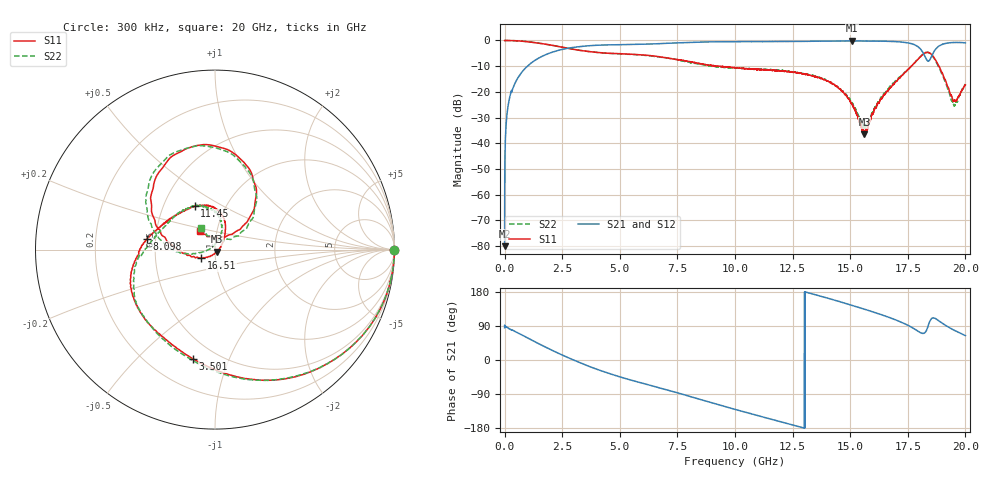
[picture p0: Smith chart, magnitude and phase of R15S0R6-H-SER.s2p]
!{R15S0R6}
!Johanson Technology Inc.
!www.johansontechnology.com
!Test Board Conditions:
!Substrate Type  RO4350B
!Substrate Thickness  20 mil
!Substrate Dk  3.66
!TL Type: GCPW
!TL Trace Width  34 mil
!TL Gap  10 mil
!Electrode orientation  Horizontal
!DUT TOPOLOGY	SERIES
!Mounting Pad LxW  26x52 mil
! Created Sat Feb  6 12:07:06 2021
# hz S ma R 50
! 2 Port Network Data from SP1.SP block
! freq  magS11  angS11  magS21  angS21  magS12  angS12  magS22  angS22
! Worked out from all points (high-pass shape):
!   20001 points, 300 kHz to 20 GHz, reference 50 ohm
!   highest |S21| = -0.15 dB at 15.06 GHz (marker M1); lowest = -80.1 dB at 300 kHz (marker M2)
!   |S21| within 3 dB of the highest: 2.681 GHz to 18.03 GHz (15.35 GHz wide, 148 % of centre); 18.73 GHz to end of sweep
!   lowest |S11| = -36.5 dB at 15.62 GHz (marker M3), VSWR 1.03, Z = 51 - j1.11 ohm
!   |S11| at or under -10 dB: 9.237 GHz to 9.311 GHz (73.82 MHz wide, 0.796 % of centre); 9.325 GHz to 17.66 GHz (8.331 GHz wide, 61.8 % of centre); 18.85 GHz to end of sweep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
!   |S22| runs from -34.1 to 0.0 dB; largest |S21 - S12| = 0.013
!   S11 on the Smith chart (normalised r, x): 300 kHz: open; 3.501 GHz: 0.38, -0.75; 8.098 GHz: 0.45, +0.06; 11.45 GHz: 0.72, +0.37; 16.51 GHz: 0.85, -0.08; 20 GHz: 0.83, +0.18
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300000  0.9962 -0.1  9.936e-05 85.0  0.0001211 68.3  0.9968 -0.2
1.013e8  0.9993 -3.5  0.03609 86.3  0.03637 86.2  0.9988 -3.5
1.343e8  0.9983 -4.6  0.04792 85.1  0.048 85.2  0.9987 -4.5
5.163e8  0.9855 -16.4  0.1676 73.4  0.1682 73.5  0.9841 -16.3
1.7933e9  0.8442 -56.4  0.5307 33.6  0.5319 33.6  0.8419 -56.2
3.3343e9  0.6358 -97.6  0.7647 -8.8  0.7658 -8.8  0.6362 -99.7
3.5013e9  0.6212 -101.4  0.7769 -12.9  0.7786 -12.9  0.6197 -104.0
6.6673e9  0.4845 -164.4  0.865 -72.7  0.867 -72.6  0.4786 -160.7
8.0983e9  0.3825 170.8  0.9168 -97.2  0.9199 -97.1  0.37 175.8
1.00003e10  0.2956 141.2  0.947 -130.3  0.9481 -130.3  0.2919 139.6
1.14483e10  0.2665 115.3  0.9516 -154.3  0.954 -154.4  0.2714 117.0
1.33343e10  0.2053 81.0  0.9652 174.8  0.9633 174.8  0.2073 89.8
1.50593e10  0.05994 42.6  0.9833 144.5  0.9781 144.7  0.06218 69.6
1.56203e10  0.01497 -46.8  0.9771 133.8  0.9745 134.3  0.02031 128.4
1.65093e10  0.08943 -149.1  0.9659 116.4  0.9637 116.2  0.09471 -167.6
1.66673e10  0.1094 -157.1  0.9652 112.8  0.9544 112.8  0.1161 -169.0
1.76383e10  0.3109 163.9  0.87 87.4  0.8635 87.3  0.3122 169.5
1.80783e10  0.4953 133.7  0.656 71.3  0.6554 71.8  0.5006 138.8
1.83343e10  0.5878 102.8  0.4107 81.5  0.4103 82.1  0.5858 105.9
1.87073e10  0.4136 56.3  0.6765 109.2  0.6781 109.1  0.3939 55.1
1.94733e10  0.06577 73.3  0.9129 79.8  0.909 80.2  0.06024 68.1
2e10  0.136 128.8  0.8982 64.3  0.8942 64.2  0.142 122.7
